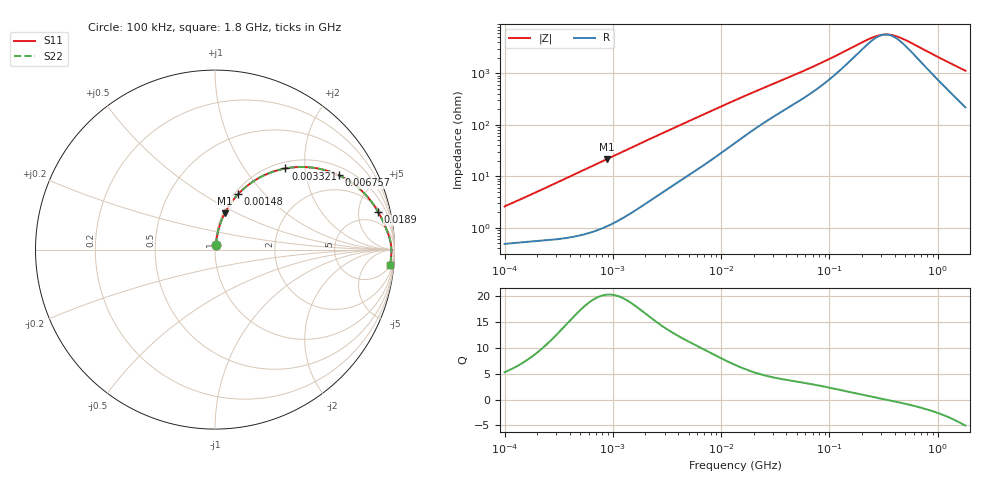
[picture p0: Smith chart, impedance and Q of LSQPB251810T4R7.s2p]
! LSQPB251810T4R7  S-PARAMETER MODEL  ( General Type )
! Model Generated by TAIYO YUDEN Corporation (http://www.ty-top.com)
! Version 2.0
! TAIYO YUDEN Control No. 100810NG22EB-FKC
! Copyright(c) 2009 TAIYO YUDEN CO.,LTD. All Rights Reserved.
! Product Description (link to TY-COMPAS)
! https://ds.yuden.co.jp/TYCOMPAS/or/detail?pn=LSQPB251810T4R7M&u=M
! Products Name : Inductors
! Characteristics :
!  Inductance : 4.7 uH , SRF(min) : 60 MHz , DC Resistance(max) : 0.429 Ohm
!  Rated Current : Saturation :650 mA , Temp Rise : 650 mA (40 degC)
!  Case Size : 2.5 x 1.8 / 0.098 x 0.071 [mm/inch] , Thickness : 1.0 / 0.04 [mm/inch]
!  (Conditions: Temperature = 25 degC , DC Bias Current/Voltage = 0A / 0V)
! External Node Assignments :
!  1  o---GGG---o  2
! GND o---------o GND
! Frequency Range : 0.1MHz  -  1800MHz  [ 402 STEP ]
# MHz S RI R 50
! Freq[MHz].  S11 Real  S11 Imag  S21 Real  S21 Imag  S12 Real  S12 Imag  S22 Real  S22 Imag
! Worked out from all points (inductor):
!   401 points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, 100 kHz to 1.8 GHz, reference 50 ohm
!   read as one part in series: L = 4.01 uH near 105 kHz
!   highest Q = 20.2 at 884.7 kHz (marker M1), where L = 3.9 uH
!   self-resonance near 329.3 MHz
!   S11 on the Smith chart (normalised r, x): 100 kHz: 1.01, +0.05; 1.48 MHz: 1.04, +0.72; 3.321 MHz: 1.12, +1.58; 6.757 MHz: 1.32, +3.11; 18.9 MHz: 2.48, +8.07; 1.8 GHz: 5, -22
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0.1  0.00547 0.0253  0.9945 -0.0253  0.9945 -0.0253  0.00547 0.0253
0.247521  0.00936 0.0604  0.9906 -0.0604  0.9906 -0.0604  0.00936 0.0604
0.516129  0.0227 0.1231  0.9773 -0.1231  0.9773 -0.1231  0.0227 0.1231
0.884704  0.054 0.2027  0.946 -0.2027  0.946 -0.2027  0.054 0.2027
1.479789  0.1277 0.3079  0.8723 -0.3079  0.8723 -0.3079  0.1277 0.3079
1.985446  0.2015 0.3722  0.7985 -0.3722  0.7985 -0.3722  0.2015 0.3722
2.66389  0.3022 0.4263  0.6978 -0.4263  0.6978 -0.4263  0.3022 0.4263
3.320932  0.3924 0.452  0.6076 -0.452  0.6076 -0.452  0.3924 0.452
4.679446  0.5431 0.4565  0.4569 -0.4565  0.4569 -0.4565  0.5431 0.4565
6.757206  0.6916 0.4135  0.3084 -0.4135  0.3084 -0.4135  0.6916 0.4135
9.52142  0.797 0.3457  0.203 -0.3457  0.203 -0.3457  0.797 0.3457
13.41641  0.867 0.2729  0.133 -0.2729  0.133 -0.2729  0.867 0.2729
18.90474  0.9098 0.2089  0.0902 -0.2089  0.0902 -0.2089  0.9098 0.2089
34.03197  0.949 0.1288  0.051 -0.1288  0.051 -0.1288  0.949 0.1288
69.24595  0.9715 0.068  0.0285 -0.068  0.0285 -0.068  0.9715 0.068
241.5136  0.9822 0.01  0.0178 -0.01  0.0178 -0.01  0.9822 0.01
301.0823  0.9826 0.00286  0.0174 -0.00286  0.0174 -0.00286  0.9826 0.00286
357.3983  0.9827 -0.00261  0.0173 0.00261  0.0173 0.00261  0.9827 -0.00261
413.9822  0.9828 -0.00737  0.0172 0.00737  0.0172 0.00737  0.9828 -0.00737
491.4156  0.9827 -0.0131  0.0173 0.0131  0.0173 0.0131  0.9827 -0.0131
1186.925  0.9801 -0.053  0.0199 0.053  0.0199 0.053  0.9801 -0.053
1800  0.9758 -0.0839  0.0242 0.0839  0.0242 0.0839  0.9758 -0.0839
